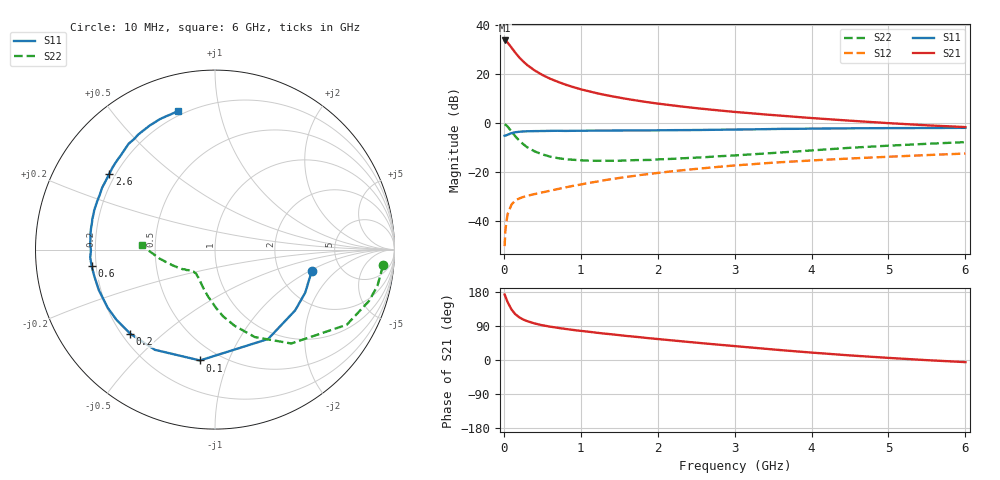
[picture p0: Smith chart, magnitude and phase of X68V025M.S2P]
! SIEMENS Small Signal Semiconductors
! BFP193W
! Si NPN RF Bipolar Junction Transistor in SOT343
! VCE = 8 V  IC = 25 mA
! Common Emitter S-Parameters:  April 1994
# GHz  S  MA  R  50
!  f  S11  S21  S12  S22
! GHz  MAG  ANG  MAG  ANG  MAG  ANG  MAG  ANG
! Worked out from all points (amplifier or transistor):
!   40 points, 10 MHz to 6 GHz, reference 50 ohm
!   highest |S21| = 33.7 dB at 10 MHz (marker M1)
!   |S21| within 3 dB of that: start of sweep to 101.9 MHz
!   unconditionally stable (mu >= 1): 934.6 MHz to 4.539 GHz
!   at 200 MHz: K = 0.38, MSG = 28.7 dB, |S12| = -30.7 dB
!   at 1.5 GHz: K = 1.10, MAG = 14.5 dB, |S12| = -22.4 dB
!   at 6 GHz: K = 0.94, MSG = 5.4 dB, |S12| = -12.4 dB
!   S11 on the Smith chart (normalised r, x): 10 MHz: 3.07, -1.05; 100 MHz: 0.39, -0.79; 200 MHz: 0.23, -0.39; 600 MHz: 0.18, -0.06; 2.6 GHz: 0.18, +0.31; 6 GHz: 0.18, +0.75
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0.01  0.5523 -12.5  48.24 172.8  0.0031 83.8  0.9405 -5.4
0.02  0.5569 -25.5  47.68 168.0  0.0064 78.3  0.9273 -12.6
0.03  0.5605 -37.2  46.65 162.6  0.0089 75.0  0.9043 -18.5
0.05  0.5793 -59.3  43.46 152.4  0.0141 66.6  0.8451 -29.7
0.1  0.6232 -97.7  34.46 133.2  0.0219 52.7  0.6741 -50.9
0.15  0.6509 -120.9  27.08 120.7  0.0266 44.7  0.5356 -65.5
0.2  0.6653 -135.2  21.77 112.7  0.0291 42.1  0.4387 -75.5
0.25  0.6741 -144.6  18.15 107.0  0.0311 40.3  0.3744 -83.1
0.3  0.6799 -151.5  15.39 102.8  0.0328 40.0  0.3239 -89.1
0.4  0.6855 -160.8  11.83 96.4  0.0357 41.2  0.2653 -98.2
0.5  0.6885 -167.5  9.582 91.7  0.0387 43.1  0.2303 -105.4
0.6  0.6932 -172.4  8.034 88.1  0.0417 45.3  0.2075 -111.1
0.8  0.6912 -179.6  6.082 82.0  0.0488 49.2  0.1838 -119.0
1.1  0.6998 172.3  4.469 74.6  0.0601 52.5  0.1712 -127.3
1.3  0.7016 167.8  3.785 69.9  0.0682 53.9  0.1708 -130.7
1.6  0.7079 161.9  3.102 63.4  0.0802 54.6  0.1723 -134.7
2.2  0.7173 151.2  2.282 51.5  0.1045 53.6  0.1868 -142.2
2.6  0.7245 144.4  1.941 43.9  0.1204 51.9  0.201 -146.9
3.2  0.7427 134.9  1.591 33.2  0.144 48.6  0.2295 -154.1
4.5  0.781 117.8  1.118 12.1  0.1896 40.3  0.3135 -170.9
5.5  0.792 109.0  0.9 -0.4  0.2226 34.2  0.3778 180.0
6  0.7985 104.8  0.828 -5.6  0.2394 31.6  0.409 176.6
